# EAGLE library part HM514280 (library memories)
DRAM 256K x 18 bits Hitachi
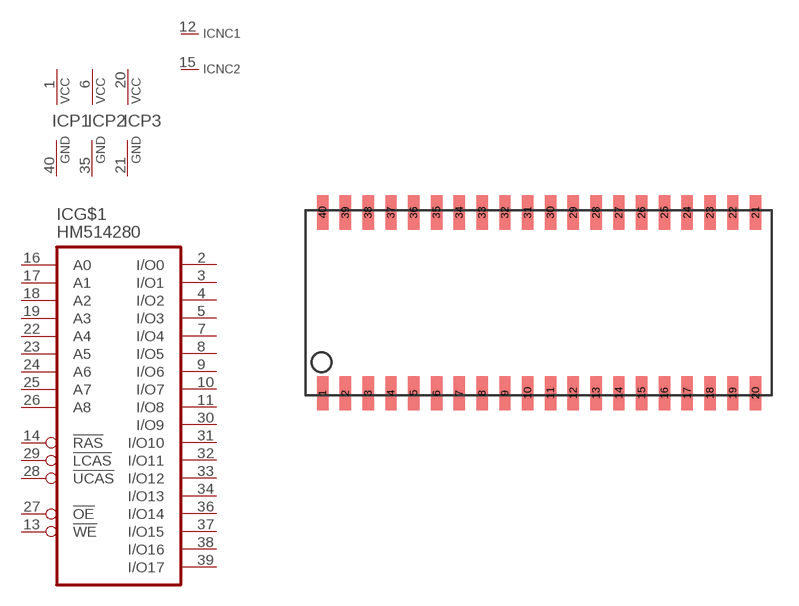
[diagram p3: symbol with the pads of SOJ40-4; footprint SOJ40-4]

Designator prefix IC; gates G$1=DRAM256KX18 P1=PWRN P2=PWRN P3=PWRN NC1=NC NC2=NC

## HM514280J  [SOJ40-4]
1  P1:VCC  pwr
2  G$1:I/O0  hiz
3  G$1:I/O1  hiz
4  G$1:I/O2  hiz
5  G$1:I/O3  hiz
6  P2:VCC  pwr
7  G$1:I/O4  hiz
8  G$1:I/O5  hiz
9  G$1:I/O6  hiz
10  G$1:I/O7  hiz
11  G$1:I/O8  hiz
12  NC1:NC  nc
13  G$1:!WE  in
14  G$1:!RAS  in
15  NC2:NC  nc
16  G$1:A0  in
17  G$1:A1  in
18  G$1:A2  in
19  G$1:A3  in
20  P3:VCC  pwr
21  P3:GND  pwr
22  G$1:A4  in
23  G$1:A5  in
24  G$1:A6  in
25  G$1:A7  in
26  G$1:A8  in
27  G$1:!OE  in
28  G$1:!UCAS  in
29  G$1:!LCAS  in
30  G$1:I/O9  hiz
31  G$1:I/O10  hiz
32  G$1:I/O11  hiz
33  G$1:I/O12  hiz
34  G$1:I/O13  hiz
35  P2:GND  pwr
36  G$1:I/O14  hiz
37  G$1:I/O15  hiz
38  G$1:I/O16  hiz
39  G$1:I/O17  hiz
40  P1:GND  pwr

## Footprint SOJ40-4 (pad centres in mm)
Small Outline J-Bend
smd 0.635 x 1.905: 1 -10.16,-5.029; 2 -8.89,-5.029; 3 -7.62,-5.029; 4 -6.35,-5.029; 5 -5.08,-5.029; 6 -3.81,-5.029; 7 -2.54,-5.029; 8 -1.27,-5.029; 9 0,-5.029; 10 1.27,-5.029; 11 2.54,-5.029; 12 3.81,-5.029; 13 5.08,-5.029; 14 6.35,-5.029; 15 7.62,-5.029; 16 8.89,-5.029; 17 10.16,-5.029; 18 11.43,-5.029; 19 12.7,-5.029; 20 13.97,-5.029; 21 13.97,5.029; 22 12.7,5.029; 23 11.43,5.029; 24 10.16,5.029; 25 8.89,5.029; 26 7.62,5.029; 27 6.35,5.029; 28 5.08,5.029; 29 3.81,5.029; 30 2.54,5.029; 31 1.27,5.029; 32 0,5.029; 33 -1.27,5.029; 34 -2.54,5.029; 35 -3.81,5.029; 36 -5.08,5.029; 37 -6.35,5.029; 38 -7.62,5.029; 39 -8.89,5.029; 40 -10.16,5.029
